TYPE DUT_material :
STRUCT
	lrLength		:	LREAL;
	lrWidth			:	LREAL;
	lrHeight		:	LREAL;
	lrArea			:	LREAL;
	lrCenterX		:	LREAL;
	lrCenterY		:	LREAL;
	lrAngle			:	LREAL;
	lrPhotoTime		:	LREAL;// Unit:s
	lrPhotoBeltPos	:	LREAL;
	bmaterial		:	BOOL;
END_STRUCT
END_TYPE
